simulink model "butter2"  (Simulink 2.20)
settings: Solver=VariableStepDiscrete  StartTime=0.0  StopTime=20.0  RelTol=1e-3  AbsTol=1e-6

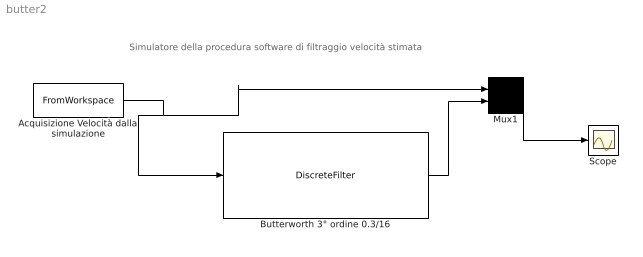
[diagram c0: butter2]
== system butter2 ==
  note: Simulatore della procedura software di filtraggio velocità stimata
  Acquisizione Velocità dalla simulazione : FromWorkspace  VariableName=[out(:,1),out(:,12)]
  Butterworth 3° ordine 0.3/16 : DiscreteFilter  Numerator="[0.0.0008    0.0017    0.0008]"  Denominator="[1.0000   -1.9167    0.9201]"  SampleTime=.033
  Mux1 : Mux  Inputs=2
  Scope : Scope
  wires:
  Mux1/1 -> Scope/1
  Acquisizione Velocità dalla simulazione/1 -> Butterworth 3° ordine 0.3/16/1, Mux1/1
  Butterworth 3° ordine 0.3/16/1 -> Mux1/2
